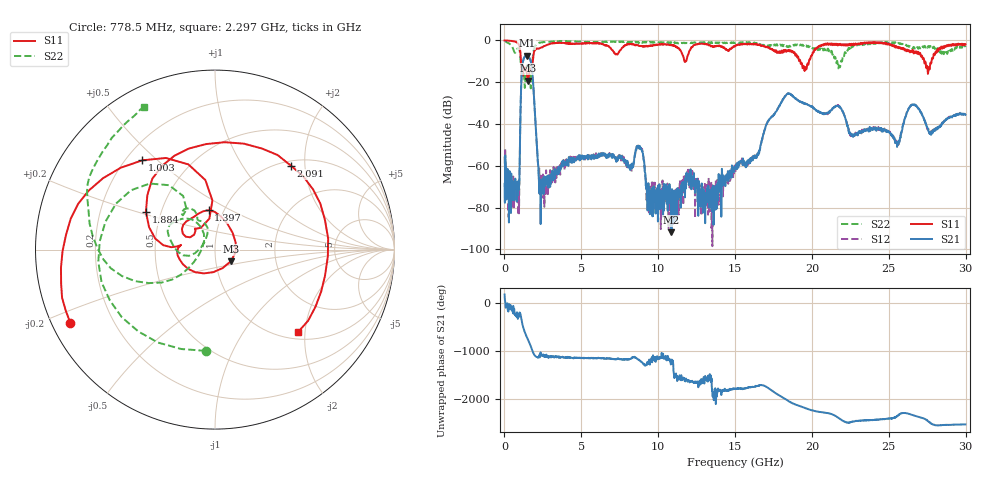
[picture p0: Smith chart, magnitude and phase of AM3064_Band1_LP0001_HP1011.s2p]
# Hz S DB R 50.0
!freq dBS11 angS11 dBS21 angS21 dBS12 angS12 dBS22 angS22
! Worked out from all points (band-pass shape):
!   1600 points, 10 MHz to 29.98 GHz, reference 50 ohm
!   highest |S21| = -7.37 dB at 1.453 GHz (marker M1); lowest = -91.9 dB at 10.86 GHz (marker M2)
!   |S21| within 3 dB of the highest: 1.197 GHz to 1.722 GHz (525.1 MHz wide, 36 % of centre)
!   lowest |S11| = -19.2 dB at 1.528 GHz (marker M3), VSWR 1.25, Z = 59.1 - j7.81 ohm
!   |S11| at or under -10 dB: 1.071 GHz to 1.839 GHz (767.9 MHz wide, 52.8 % of centre); 19.24 GHz to 19.8 GHz (559.7 MHz wide, 2.87 % of centre); 27.3 GHz to 27.78 GHz (479.6 MHz wide, 1.74 % of centre)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
!   |S22| runs from -23.0 to -0.2 dB; largest |S21 - S12| = 0.005
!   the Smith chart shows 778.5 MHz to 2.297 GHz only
!   S11 on the Smith chart (normalised r, x): 778.5 MHz: 0.05, -0.24; 1.003 GHz: 0.26, +0.45; 1.397 GHz: 0.85, +0.39; 1.884 GHz: 0.41, +0.21; 2.091 GHz: 1.10, +1.70; 2.297 GHz: 1.14, -1.83
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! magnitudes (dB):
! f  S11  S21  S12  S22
! 10 MHz  0.0  -68.6  -55.6  -0.2
! 778.5 MHz  -0.9  -67.8  -73.5  -4.9
! 1.003 GHz  -3.9  -51.6  -51.6  -5.7
! 1.191 GHz  -16.9  -10.6  -10.6  -13.8
! 1.397 GHz  -13.1  -7.4  -7.4  -14.8
! 1.453 GHz  -15.9  -7.4  -7.3  -12.0
! 1.528 GHz  -19.2  -7.6  -7.5  -10.8
! 1.884 GHz  -7.2  -22.6  -22.6  -5.4
! 2.091 GHz  -4.0  -48.3  -48.6  -1.8
! 2.297 GHz  -3.7  -66.6  -66.0  -1.1
! 5.015 GHz  -1.4  -55.6  -56.8  -0.7
! 8.801 GHz  -2.6  -51.3  -51.1  -1.0
! 9.401 GHz  -2.5  -74.1  -83.1  -0.8
! 10 GHz  -2.0  -70.7  -77.4  -0.9
! 10.86 GHz  -2.4  -91.9  -81.4  -1.2
! 15 GHz  -2.7  -60.3  -60.8  -1.2
! 18.36 GHz  -5.2  -25.7  -25.9  -3.0
! 19.99 GHz  -7.3  -31.9  -31.8  -3.3
! 25 GHz  -1.5  -43.5  -43.7  -1.2
! 26.59 GHz  -5.3  -30.6  -30.7  -3.4
! 27.56 GHz  -15.1  -43.1  -42.8  -2.8
! 29.98 GHz  -1.8  -35.6  -35.5  -3.2
